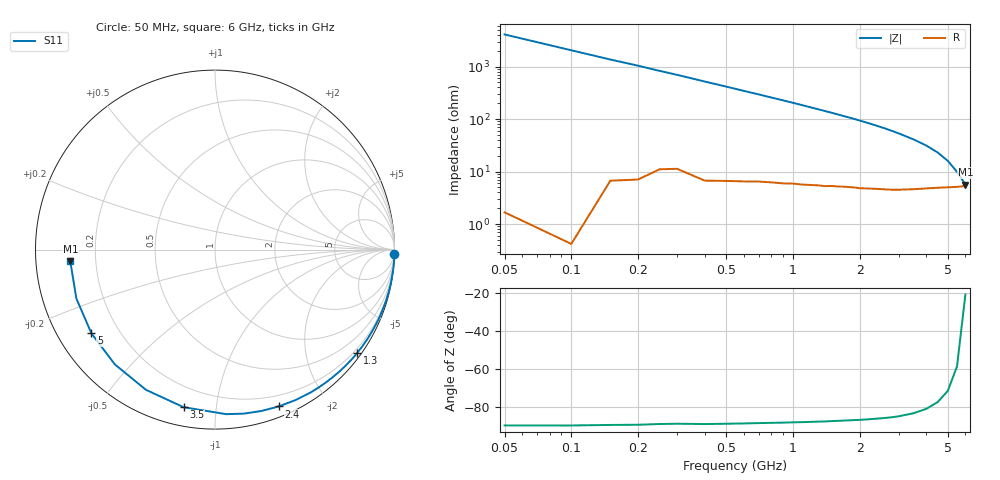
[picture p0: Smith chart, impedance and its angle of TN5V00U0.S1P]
! SIEMENS Discrete & RF Semiconductors
! BAS70-07W
! Si Schottky Diode in SOT343
! VR = 5 V
! S-Parameters:  February  1997
# GHz  S  MA  R  50
!  f  S11
! GHz  MAG  ANG
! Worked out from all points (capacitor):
!   34 points, 50 MHz to 6 GHz, reference 50 ohm
!   read as one part to ground: C = 778 fF near 50 MHz
!   lowest |Z| = 5.67 ohm at 6 GHz (marker M1)
!   S11 on the Smith chart (normalised r, x): 50 MHz: 0, -82; 1.3 GHz: 0.11, -3.07; 2.4 GHz: 0.09, -1.48; 3.5 GHz: 0.09, -0.82; 5 GHz: 0.10, -0.30; 6 GHz: 0.11, -0.04
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0.05  1 -1.4
0.15  0.9996 -4.2
0.2  0.9993 -5.5
0.4  0.9975 -11.0
0.5  0.9962 -13.7
0.6  0.9947 -16.5
0.7  0.9928 -19.2
0.8  0.991 -22.0
0.9  0.9891 -24.7
1.1  0.9846 -30.3
1.2  0.982 -33.2
1.3  0.9793 -36.0
1.4  0.9769 -38.8
1.6  0.9706 -44.5
1.7  0.9672 -47.4
1.8  0.9641 -50.2
2  0.9583 -56.0
2.2  0.9508 -61.9
2.4  0.9431 -67.9
2.6  0.9357 -73.9
2.8  0.9279 -80.0
3  0.919 -86.1
3.5  0.8952 -101.3
4  0.8708 -116.2
4.5  0.8487 -131.1
5  0.8318 -145.9
5.5  0.819 -160.6
6  0.8087 -175.3
